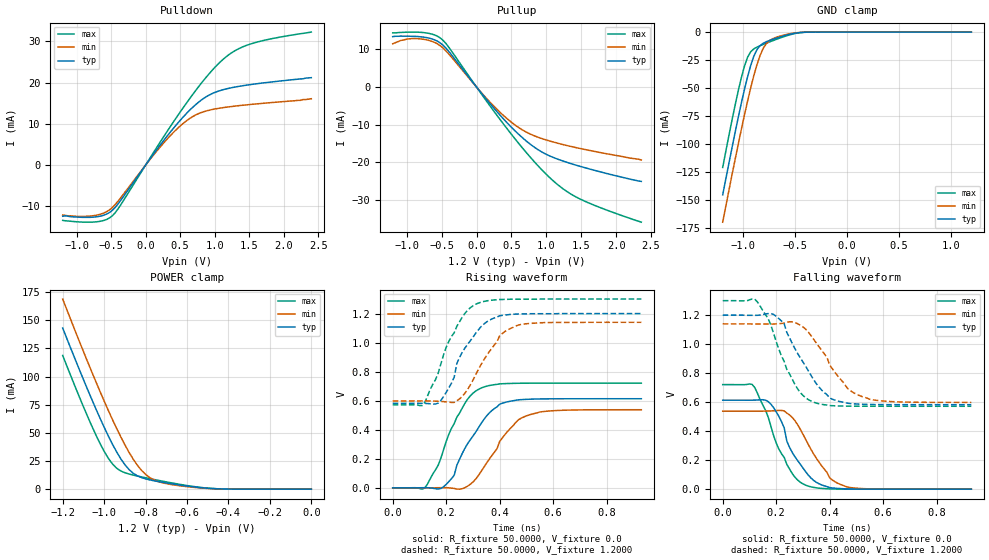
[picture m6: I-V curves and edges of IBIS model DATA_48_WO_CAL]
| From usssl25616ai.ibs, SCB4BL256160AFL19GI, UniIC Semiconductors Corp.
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|   Model DATA_48_WO_CAL
[Model]  DATA_48_WO_CAL
Model_type I/O
Polarity   Non-Inverting
Enable   Active-High
Vinl =   0.3800V
Vinh =   0.8200V
Vmeas =  0.6000V
Cref =   5.0000pF
Rref =   50.0000
Vref =   0.6000V
C_comp   1.7430pF   1.7110pF   1.7640pF
[Temperature Range]   25.0000   85.0000   -40.0000
[Voltage Range]   1.2000V   1.1400V   1.3000V
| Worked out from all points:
|   slope of the pulldown table from 0 to 0.18 V, typ, clamps not added: 43.4 ohm
|   slope of the pullup table from 0 to 0.18 V, typ, clamps not added: 43.8 ohm
|   GND clamp passes 1 mA (typ) near -0.50 V on its own axis
|   POWER clamp passes 1 mA (typ) near -0.51 V on its own axis
|   rising waveform, R_fixture 50.0000, V_fixture 0.0: 20-80 % time 114ps typ, 123ps min, 102ps max; typ from 0 V to 0.614 V
|   rising waveform, R_fixture 50.0000, V_fixture 1.2000: 20-80 % time 100ps typ, 106ps min, 102ps max; typ from 0.582 V to 1.2 V
|   falling waveform, R_fixture 50.0000, V_fixture 0.0: 20-80 % time 96.3ps typ, 108ps min, 97.3ps max; typ from 0.614 V to 0 V
|   falling waveform, R_fixture 50.0000, V_fixture 1.2000: 20-80 % time 118ps typ, 121ps min, 97ps max; typ from 1.2 V to 0.582 V
[Pulldown]
|Voltage   I(typ)   I(min)   I(max)
-1.2V     -12.4mA    -12.1mA    -13.4mA
-760mV    -12.61mA   -12.27mA   -13.81mA
-600mV    -12.12mA   -11.59mA   -13.4mA
-480mV    -10.93mA   -10.25mA   -12.26mA
-360mV    -8.541mA   -7.918mA   -9.637mA
200mV     4.598mA    4.169mA    5.291mA
520mV     11.21mA    9.771mA    13.33mA
840mV     16.17mA    12.94mA    20.55mA
1.2V      18.61mA    14.12mA    26.7mA
1.4V      19.23mA    14.51mA    28.63mA
1.6V      19.72mA    14.84mA    29.77mA
2.4V      21.2mA     16.1mA     32.26mA
[Pullup]
|Voltage   I(typ)   I(min)   I(max)
-1.2V     13.4mA     11.5mA     14.4mA
-880mV    13.47mA    12.89mA    14.6mA
-680mV    13.01mA    12.39mA    14.26mA
-520mV    11.74mA    11mA       13.06mA
-400mV    9.531mA    8.844mA    10.66mA
320mV     -7.122mA   -6.417mA   -8.209mA
560mV     -11.8mA    -10.22mA   -13.98mA
840mV     -16.16mA   -13.07mA   -20.12mA
1.12V     -18.88mA   -14.73mA   -25.3mA
1.4V      -20.64mA   -16.01mA   -28.99mA
1.76V     -22.5mA    -17.39mA   -31.99mA
2.36V     -25.1mA    -19.4mA    -35.95mA
[GND_clamp]
|Voltage   I(typ)   I(min)   I(max)
-1.2V     -145.3mA   -169.7mA   -120.8mA
-1.11V    -103.1mA   -127.3mA   -78.51mA
-1.05V    -76.2mA    -100.1mA   -52.43mA
-990mV    -51.2mA    -74mA      -30.39mA
-960mV    -39.9mA    -61.63mA   -22.48mA
-900mV    -21.67mA   -39mA      -15mA
-870mV    -15.78mA   -29.25mA   -13.45mA
-810mV    -10.04mA   -14.72mA   -11.07mA
-750mV    -7.557mA   -7.71mA    -8.865mA
-600mV    -3.111mA   -2.463mA   -3.804mA
-420mV    -215.4uA   -156.1uA   -235uA
1.2V      1.597nA    5.589nA    1.463nA
[POWER_clamp]
|Voltage   I(typ)   I(min)   I(max)
-1.2V     143mA      168.8mA    118.7mA
-1.06V    79.88mA    104.3mA    56.26mA
-1.02V    63.08mA    86.79mA    40.63mA
-980mV    47.32mA    69.97mA    27.48mA
-940mV    33.2mA     54.05mA    18.67mA
-880mV    17.43mA    32.78mA    13.45mA
-840mV    11.87mA    21.34mA    11.69mA
-800mV    9.133mA    13.1mA     10.12mA
-720mV    6.135mA    5.731mA    7.166mA
-560mV    1.838mA    1.456mA    2.161mA
-420mV    156.9uA    132.7uA    153uA
0V        1.597nA    1.927nA    2.16nA
[Ramp]
| variable   typ   min   max
dV/dt_r  0.3682/0.1099n   0.3228/0.1239n   0.4326/0.1041n
dV/dt_f  0.3705/0.1101n   0.3249/0.1275n   0.4370/99.4795p
R_load = 50.0000
[Rising Waveform]
R_fixture= 50.0000
V_fixture= 0.0
V_fixture_min= 0.0
V_fixture_max= 0.0
|time   V(typ)   V(min)   V(max)
0s        0V         0V         0V
120ps     1.127mV    198uV      -350.4uV
170ps     -8.205mV   1.014mV    155.4mV
220ps     63.52mV    -1.813mV   410.3mV
280ps     303.9mV    11.58mV    610.2mV
330ps     441.1mV    110.7mV    686.6mV
400ps     575.9mV    318.9mV    715.9mV
470ps     606mV      468.7mV    720.2mV
500ps     609.5mV    495.5mV    720.6mV
930ps     613.7mV    538mV      721mV
[Rising Waveform]
R_fixture= 50.0000
V_fixture= 1.2000
V_fixture_min= 1.1400
V_fixture_max= 1.3000
|time   V(typ)   V(min)   V(max)
0s        582.5mV    598.5mV    571.7mV
110ps     582.1mV    598.9mV    566.6mV
170ps     583.7mV    596.3mV    788.8mV
200ps     657.6mV    592mV      967.5mV
220ps     721.7mV    588.3mV    1.043V
250ps     898.1mV    612.4mV    1.144V
320ps     1.087V     813.2mV    1.272V
400ps     1.185V     1.047V     1.297V
470ps     1.197V     1.121V     1.299V
930ps     1.2V       1.14V      1.3V
[Falling Waveform]
R_fixture= 50.0000
V_fixture= 0.0
V_fixture_min= 0.0
V_fixture_max= 0.0
|time   V(typ)   V(min)   V(max)
0s        613.7mV    538mV      721mV
110ps     613.6mV    537.6mV    722.3mV
170ps     603.9mV    538.8mV    498mV
200ps     534.4mV    541.8mV    318.8mV
220ps     465mV      542.6mV    244.3mV
240ps     330.5mV    524.6mV    170.6mV
310ps     120.9mV    344.3mV    27.87mV
400ps     10.85mV    78.23mV    1.752mV
460ps     2.161mV    18.62mV    291uV
930ps     0V         0V         0V
[Falling Waveform]
R_fixture= 50.0000
V_fixture= 1.2000
V_fixture_min= 1.1400
V_fixture_max= 1.3000
|time   V(typ)   V(min)   V(max)
0s        1.2V       1.14V      1.3V
130ps     1.199V     1.139V     1.291V
170ps     1.211V     1.139V     1.176V
230ps     1.14V      1.145V     880.7mV
280ps     936.5mV    1.141V     692.3mV
340ps     755.6mV    1.034V     600.1mV
400ps     629mV      856.9mV    576.8mV
470ps     591.8mV    688.9mV    572.4mV
510ps     586.6mV    646.8mV    572mV
930ps     582.5mV    598.5mV    571.7mV
